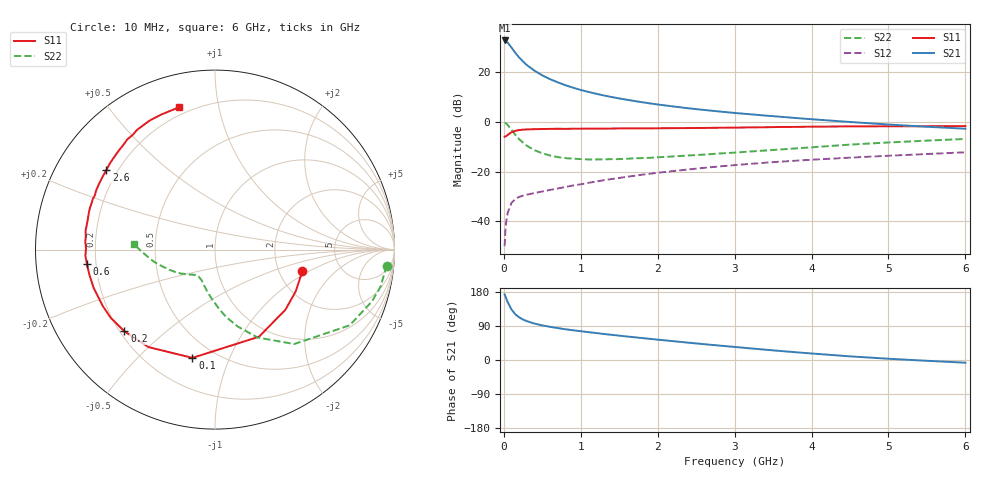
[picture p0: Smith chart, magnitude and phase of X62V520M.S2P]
! SIEMENS Small Signal Semiconductors
! BFP193W
! Si NPN RF Bipolar Junction Transistor in SOT343
! VCE = 2.5 V  IC = 20 mA
! Common Emitter S-Parameters:  April 1994
# GHz  S  MA  R  50
!  f  S11  S21  S12  S22
! GHz  MAG  ANG  MAG  ANG  MAG  ANG  MAG  ANG
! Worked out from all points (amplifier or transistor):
!   40 points, 10 MHz to 6 GHz, reference 50 ohm
!   highest |S21| = 32.6 dB at 10 MHz (marker M1)
!   |S21| within 3 dB of that: start of sweep to 102.9 MHz
!   unconditionally stable (mu >= 1): 935.7 MHz to 3.979 GHz
!   at 200 MHz: K = 0.36, MSG = 27.9 dB, |S12| = -30.1 dB
!   at 1.5 GHz: K = 1.11, MAG = 13.9 dB, |S12| = -22.5 dB
!   at 6 GHz: K = 0.93, MSG = 4.7 dB, |S12| = -12.3 dB
!   lowest NFmin = 1.40 dB at 450 MHz
!   S11 on the Smith chart (normalised r, x): 10 MHz: 2.70, -0.86; 100 MHz: 0.38, -0.74; 200 MHz: 0.22, -0.37; 600 MHz: 0.16, -0.06; 2.6 GHz: 0.16, +0.32; 6 GHz: 0.16, +0.77
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0.01  0.5017 -13.7  42.56 173.3  0.0032 86.9  0.9605 -5.3
0.02  0.5063 -27.4  42.16 168.3  0.0066 79.3  0.9455 -12.5
0.03  0.516 -40.5  41.32 162.8  0.0097 76.6  0.9212 -18.2
0.05  0.5437 -63.2  38.53 152.5  0.0149 67.1  0.8612 -29.3
0.1  0.6163 -101.8  30.55 133.2  0.0236 51.3  0.6869 -50.0
0.15  0.6575 -124.3  24.03 120.5  0.0285 43.7  0.5447 -64.1
0.2  0.6796 -137.9  19.31 112.5  0.0311 40.2  0.4463 -73.6
0.25  0.6945 -146.8  16.1 106.7  0.033 38.2  0.3801 -80.7
0.3  0.6999 -153.4  13.64 102.4  0.0345 37.8  0.3289 -86.3
0.4  0.7089 -162.4  10.49 96.0  0.0372 38.6  0.2685 -94.8
0.5  0.714 -168.8  8.501 91.3  0.0399 40.6  0.2332 -101.3
0.6  0.7178 -173.5  7.125 87.5  0.0429 42.4  0.2103 -106.4
0.8  0.7185 179.4  5.396 81.2  0.0492 46.7  0.1865 -113.7
1.1  0.7289 171.8  3.964 73.5  0.0595 50.5  0.1752 -121.3
1.3  0.7281 167.1  3.359 68.7  0.0672 52.1  0.1763 -124.7
1.6  0.7345 161.3  2.755 62.0  0.0787 53.4  0.1807 -128.7
2.2  0.7427 150.6  2.025 49.7  0.1025 53.5  0.2011 -136.7
2.6  0.7499 143.8  1.723 41.8  0.1187 52.2  0.2188 -142.0
3.2  0.7686 134.4  1.412 30.8  0.1428 49.3  0.2528 -150.2
4.5  0.8057 117.0  0.988 9.6  0.1905 41.3  0.3476 -168.9
5.5  0.8118 108.2  0.793 -2.1  0.2253 35.1  0.4183 -179.7
6  0.8179 104.2  0.724 -7.1  0.2439 32.4  0.4514 176.2
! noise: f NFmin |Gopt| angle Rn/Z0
0.45  1.4  0.3  160  0.1
0.9  1.45  0.34  172  0.11
1.8  2.2  0.56  -148  0.2
